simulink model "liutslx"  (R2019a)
settings: configuration reference "configurationSettings" (kept in a data dictionary, not in this file)
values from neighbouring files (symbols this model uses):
  ag = NaN(L.ng,1)    [bdet.m]
  D = meqp()    [fbtp.m]
  dr2FA = dr2Fs(1:nA,1)    [asxycs.m]
  drzFA = drzFs(1:nA,1)    [asxycs.m]
  dz = dzxs(is)    [asxycsJac.m]    (also in bintc.m = (z - zx(kz))/dzx)
  dz2FA = dz2Fs(1:nA,1)    [asxycs.m]
  err = [IaeH            ; IoeH               ; IueH               ; DeH               ; FeH            ; BeH               ; BeH               ; BeH               ; CeH               ; CeH               ; CeH               ; VeH                ; VeH                ; VeH               ]    [fbtopt.m]
  FA = Fs(1:nA,1)    [asxycs.m]    (also in bfhelp.m = [-1                        0        0       ])
  FB = [0                         1        1       ]    [bfhelp.m]
  Fx = meqFx(L,Iy,[Ia;Iu])    [bdet.m]    (also in bfhelp.m = zeros(n+2,3); Fx(2:end-1,2) = FN)
  FX = Fs(nA+1:ns,1)    [asxycs.m]
  Iy = LXt.Iy    [bdet.m]    (also in fbtinit.m = meqinitIy(L,LXs.t,IpD,bbs,LXs.capaj))
  L = fbtc(P,G)    [fbt.m]    (also in fbtc.m = meqc(P,G); fbte.m = varargout{1})
  nA = numel(rA)    [asxycs.m]
  niter = L.P.itercs    [asxycs.m]
  Opy = logical(Opy)    [bfct.m]    (also in bfdoublet.m = Opy==1 | Opy==2)
  rA = rs(1:nA,1)    [asxycs.m]    (also in fbtptcv.m = (rA1 + 3*rA2)/4)
  rX = rs(nA+1:ns,1)    [asxycs.m]    (also in fbtptcv.m = rzbro(iX,1); fbtxana.m = r0)
  zA = zs(1:nA,1)    [asxycs.m]    (also in fbtptcv.m = (zA1 + 3*zA2)/4)
  zX = zs(nA+1:ns,1)    [asxycs.m]    (also in fbtptcv.m = rzbro(iX,2); fbtxana.m = 0)
undefined symbols (not defined in the file or in its folder): Bm, bp, bpli2, Brn, Brrn, Brzn, bt, Bzn, Bzrn, Bzzn, dzg, Ff, Fn, Ft, Ft0, Ie, Ip, iTQ, lB, li, lX, mu, nX, PpQ, PQ, rB, rBt, repmat, Row, rst, TQ, TTpQ, Un, vector, Vp, Wk, WN, Wp, Wt, Wt0, zB
libraries: liulib x34, mkllib x28, simulink x5
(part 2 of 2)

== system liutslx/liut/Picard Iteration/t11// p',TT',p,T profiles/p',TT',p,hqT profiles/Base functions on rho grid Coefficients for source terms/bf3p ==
  ag : Inport
  FA : Inport  Port=2
  FB : Inport  Port=3
  fPg : Inport  Port=4
  fTg : Inport  Port=5
  BF3P3 : liulib/BF3P3  idsx=L.idsx
  Terminator1 : Terminator
  Terminator2 : Terminator
  aPpg : Outport
  aTTpg : Outport  Port=2
  aPg : Outport  Port=3
  ahqTg : Outport  Port=4
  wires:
  fPg/1 -> Terminator2/1
  fTg/1 -> Terminator1/1
  ag/1 -> BF3P3/1
  FA/1 -> BF3P3/2
  FB/1 -> BF3P3/3
  BF3P3/1 -> aPpg/1
  BF3P3/2 -> aTTpg/1
  BF3P3/3 -> aPg/1
  BF3P3/4 -> ahqTg/1

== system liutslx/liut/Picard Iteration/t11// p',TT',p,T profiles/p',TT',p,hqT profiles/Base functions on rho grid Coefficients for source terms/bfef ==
  ag : Inport
  FA : Inport  Port=2
  FB : Inport  Port=3
  fPg : Inport  Port=4
  fTg : Inport  Port=5
  BFEF3 : liulib/BFEF3  ids=L.idsx  nP=L.P.bfp(1)  nT=L.P.bfp(2)
  Terminator : Terminator
  Terminator1 : Terminator
  aPpg : Outport
  aTTpg : Outport  Port=2
  aPg : Outport  Port=3
  ahqTg : Outport  Port=4
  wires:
  fTg/1 -> Terminator1/1
  fPg/1 -> Terminator/1
  BFEF3/4 -> ahqTg/1
  BFEF3/3 -> aPg/1
  BFEF3/2 -> aTTpg/1
  BFEF3/1 -> aPpg/1
  FB/1 -> BFEF3/3
  FA/1 -> BFEF3/2
  ag/1 -> BFEF3/1
